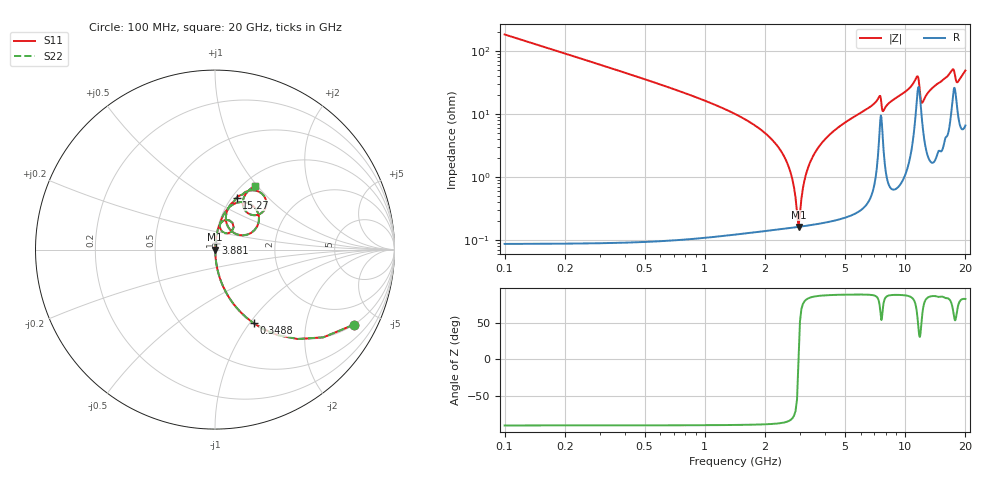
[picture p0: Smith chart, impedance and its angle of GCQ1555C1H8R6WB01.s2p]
!Murata Part Number: GCQ1555C1H8R6WB01
!These Parameters are Measured in Series Mode Connection
!Data Generated on Mar 13, 2026
!  o--ll--o
!Port1  Port2
!  o------o
!Operation Temp=25[degC], DC Bias Voltage=0[V]
!Freq. Start=100[MHz] Stop=20[GHz] 401[Steps]
# Hz S RI R 50
!Freq.(Hz) S11(Real) S11(Imag) S21(Real) S21(Imag) S12(Real) S12(Imag) S22(Real) S22(Imag)
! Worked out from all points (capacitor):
!   401 points, 100 MHz to 20 GHz, reference 50 ohm
!   read as one part in series: C = 8.6 pF near 199.5 MHz
!   lowest |Z| = 161 mohm at 2.936 GHz (marker M1)
!   series resonance near 2.937 GHz, so ESL is about 340 pH
!   S11 on the Smith chart (normalised r, x): 100 MHz: 1.00, -3.70; 348.8 MHz: 1.00, -1.05; 3.881 GHz: 1.00, +0.07; 15.27 GHz: 1.05, +0.68; 20 GHz: 1.13, +0.98
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1e8  0.7735 -0.4183  0.2265 0.4183  0.2265 0.4183  0.7735 -0.4183
3.4875e8  0.2153 -0.4102  0.7847 0.4102  0.7847 0.4102  0.2153 -0.4102
8.4625e8  0.0396 -0.1924  0.9604 0.1924  0.9604 0.1924  0.0396 -0.1924
2.33875e9  0.0023 -0.029  0.9977 0.029  0.9977 0.029  0.0023 -0.029
2.63725e9  0.00172 -0.0136  0.9983 0.0136  0.9983 0.0136  0.00172 -0.0136
2.93575e9  0.0016 -5.77e-05  0.9984 5.77e-05  0.9984 5.77e-05  0.0016 -5.77e-05
3.1845e9  0.00177 0.0103  0.9982 -0.0103  0.9982 -0.0103  0.00177 0.0103
3.43325e9  0.00212 0.0199  0.9979 -0.0199  0.9979 -0.0199  0.00212 0.0199
3.881e9  0.00315 0.0361  0.9969 -0.0361  0.9969 -0.0361  0.00315 0.0361
4.92575e9  0.00714 0.07  0.9929 -0.07  0.9929 -0.07  0.00714 0.07
6.7665e9  0.0223 0.1303  0.9777 -0.1303  0.9777 -0.1303  0.0223 0.1303
7.463e9  0.0815 0.1619  0.9185 -0.1619  0.9185 -0.1619  0.0815 0.1619
7.81125e9  0.0366 0.1045  0.9634 -0.1045  0.9634 -0.1045  0.0366 0.1045
1.005e10  0.0592 0.2129  0.9408 -0.2129  0.9408 -0.2129  0.0592 0.2129
1.149275e10  0.2291 0.2243  0.7709 -0.2243  0.7709 -0.2243  0.2291 0.2243
1.21395e10  0.0876 0.1074  0.9124 -0.1074  0.9124 -0.1074  0.0876 0.1074
1.338325e10  0.0699 0.2214  0.9301 -0.2214  0.9301 -0.2214  0.0699 0.2214
1.527375e10  0.1211 0.2897  0.8789 -0.2897  0.8789 -0.2897  0.1211 0.2897
1.67165e10  0.2005 0.3302  0.7995 -0.3302  0.7995 -0.3302  0.2005 0.3302
1.746275e10  0.286 0.2592  0.714 -0.2592  0.714 -0.2592  0.286 0.2592
1.81095e10  0.178 0.2074  0.822 -0.2074  0.822 -0.2074  0.178 0.2074
2e10  0.2251 0.3557  0.7749 -0.3557  0.7749 -0.3557  0.2251 0.3557
